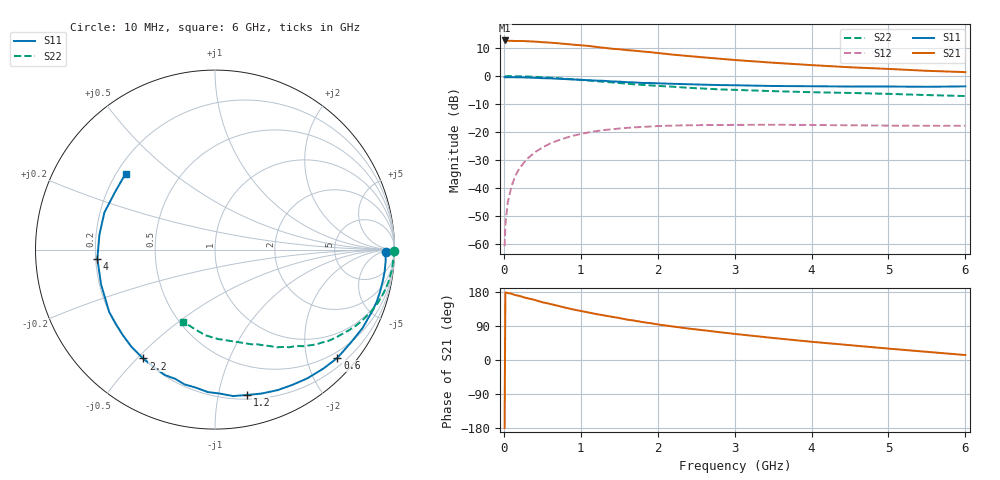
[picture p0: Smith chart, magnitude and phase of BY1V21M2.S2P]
! SIEMENS Small Signal Semiconductors
! BFY420
! Si NPN RF SIEGET Grounded Emitter Transistor in MICRO-X
! VCE = 1.25 V  IC = 1.2 mA
! Common Emitter S-Parameters:  October  1996
# GHz  S  MA  R  50
!  f  S11  S21  S12  S22
! GHz  MAG  ANG  MAG  ANG  MAG  ANG  MAG  ANG
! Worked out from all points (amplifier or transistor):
!   36 points, 10 MHz to 6 GHz, reference 50 ohm
!   highest |S21| = 12.7 dB at 10 MHz (marker M1)
!   |S21| within 3 dB of that: start of sweep to 1.423 GHz
!   unconditionally stable (mu >= 1): 4.41 GHz to end of sweep
!   at 250 MHz: K = 0.05, MSG = 22.0 dB, |S12| = -31.4 dB
!   at 1.4 GHz: K = 0.24, MSG = 14.4 dB, |S12| = -19.1 dB
!   at 6 GHz: K = 1.33, MAG = 6.2 dB, |S12| = -17.8 dB
!   S11 on the Smith chart (normalised r, x): 10 MHz: 38, -11; 600 MHz: 0.37, -2.59; 1.2 GHz: 0.23, -1.22; 2.2 GHz: 0.20, -0.52; 4 GHz: 0.21, -0.04; 6 GHz: 0.24, +0.35
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0.01  0.9523 -0.8  4.34 -179.4  0.0009 99.5  0.9988 -0.3
0.02  0.9496 -1.6  4.304 178.6  0.0022 80.8  0.9907 -0.7
0.05  0.953 -3.6  4.26 176.8  0.0054 84.4  0.997 -1.9
0.1  0.9531 -7.3  4.272 174.9  0.0107 84.8  0.9942 -3.7
0.15  0.9511 -10.5  4.237 171.1  0.0164 82.4  0.9926 -5.6
0.2  0.9492 -14.3  4.247 169.2  0.0219 82.3  0.99 -7.4
0.25  0.9466 -17.7  4.24 166.1  0.027 78.2  0.9853 -9.2
0.4  0.931 -28.0  4.139 158.7  0.0428 73.1  0.9691 -14.7
0.5  0.9165 -34.8  4.044 152.5  0.0525 68.9  0.9539 -18.3
0.6  0.9106 -41.5  3.965 148.0  0.0619 64.9  0.9369 -21.6
0.9  0.8684 -60.2  3.652 133.4  0.0855 53.2  0.8739 -30.7
1.1  0.8428 -72.1  3.465 125.4  0.0979 46.8  0.8311 -36.3
1.2  0.8295 -77.5  3.328 121.3  0.1034 43.8  0.8103 -38.9
1.6  0.7762 -98.0  2.916 106.7  0.1181 33.1  0.731 -47.4
2  0.7417 -116.1  2.587 93.9  0.1272 24.5  0.6664 -54.4
2.2  0.7265 -123.4  2.418 88.4  0.1299 20.7  0.6444 -57.6
2.8  0.6903 -143.3  2.048 73.5  0.1332 12.5  0.5777 -66.0
3.5  0.6638 -163.0  1.733 58.1  0.1345 5.7  0.5369 -74.6
4  0.6575 -175.6  1.57 48.1  0.133 2.0  0.5138 -81.2
4.5  0.6493 172.6  1.437 39.1  0.1312 -0.8  0.4985 -88.1
5.5  0.6427 150.0  1.242 21.5  0.1289 -3.7  0.4568 -104.4
6  0.6538 139.6  1.176 13.1  0.1285 -3.6  0.4389 -113.8
